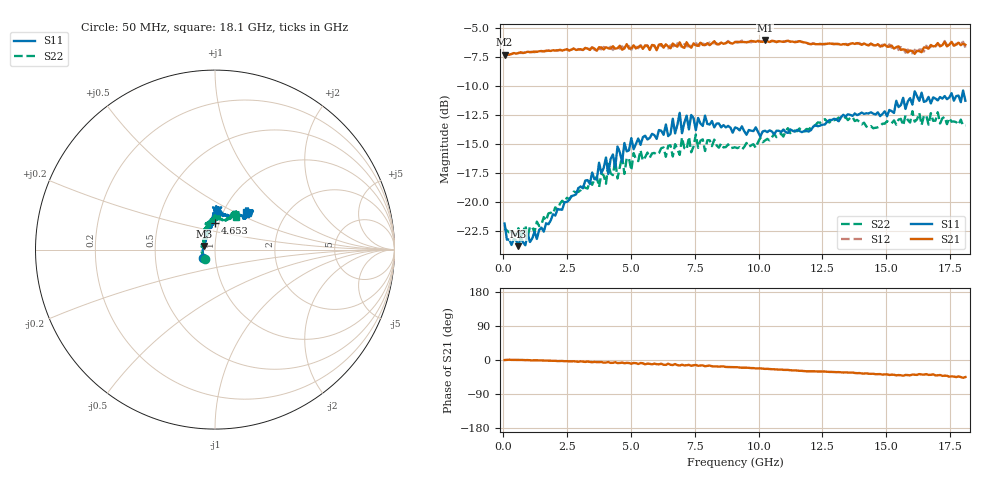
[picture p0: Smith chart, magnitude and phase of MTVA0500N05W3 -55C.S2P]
! Network Analyzer HP8720D.06.14 Serial No. US36140669
!  8 Jul 2005  09:03:04
! Frequency  S11  S21  S12  S22
# HZ  S  DB R 50
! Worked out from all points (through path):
!   201 points, 50 MHz to 18.1 GHz, reference 50 ohm
!   highest |S21| = -6.06 dB at 10.25 GHz (marker M1); lowest = -7.3 dB at 50 MHz (marker M2)
!   group delay of S21, straight-line fit = 7.47 ps
!   lowest |S11| = -23.8 dB at 591.5 MHz (marker M3), VSWR 1.14, Z = 44.2 + j1.82 ohm
!   |S11| at or under -10 dB: start of sweep to end of sweep
!   |S22| runs from -23.1 to -12.2 dB; largest |S21 - S12| = 0.025
!   S11 on the Smith chart (normalised r, x): 50 MHz: 0.87, -0.08; 4.653 GHz: 0.95, +0.29; 18.1 GHz: 1.27, +0.58
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5e7  -21.85 -145.7  -7.29 -0.1  -7.33 -0.2  -22.28 -135.2
5.915e8  -23.80 161.5  -7.15 0.0  -7.14 0.1  -22.25 167.1
9.525e8  -22.69 149.9  -7.03 -0.2  -7.10 -0.2  -23.04 154.5
3.1185e9  -18.81 107.4  -6.88 -4.2  -6.89 -4.6  -18.65 119.3
4.021e9  -16.16 100.0  -6.65 -6.7  -6.80 -5.6  -18.41 110.3
4.382e9  -17.01 96.0  -6.77 -5.9  -6.67 -7.7  -16.43 109.2
4.47225e9  -15.21 90.8  -6.74 -8.1  -6.65 -6.3  -17.96 112.5
4.65275e9  -16.53 90.7  -6.87 -6.8  -6.57 -7.9  -16.04 110.8
4.743e9  -14.91 93.3  -6.75 -8.5  -6.76 -7.2  -17.57 106.7
5.104e9  -15.45 95.2  -6.48 -7.8  -6.53 -9.2  -15.77 101.7
6.09675e9  -13.79 88.2  -6.42 -11.5  -6.37 -11.2  -15.77 97.7
6.7285e9  -14.07 92.2  -6.49 -10.6  -6.74 -12.2  -15.00 90.8
6.909e9  -12.30 88.6  -6.22 -14.4  -6.46 -12.7  -15.93 89.1
6.99925e9  -14.06 88.4  -6.61 -12.5  -6.66 -14.7  -14.43 89.9
7.36025e9  -12.49 81.6  -6.69 -15.1  -6.44 -13.5  -15.70 93.4
7.54075e9  -13.80 83.1  -6.49 -13.0  -6.28 -15.6  -14.17 92.0
9.075e9  -13.56 84.3  -6.21 -18.9  -6.18 -18.9  -15.28 78.5
1.024825e10  -13.85 78.6  -6.06 -23.5  -6.17 -23.3  -14.69 63.9
1.21435e10  -13.48 65.1  -6.34 -29.7  -6.30 -29.8  -13.47 65.6
1.512175e10  -12.06 45.6  -6.59 -39.5  -6.40 -38.9  -13.16 61.9
1.61145e10  -10.45 45.2  -7.21 -38.9  -6.87 -38.6  -13.07 61.1
1.81e10  -11.26 50.6  -6.44 -45.0  -6.68 -45.8  -13.39 57.5
